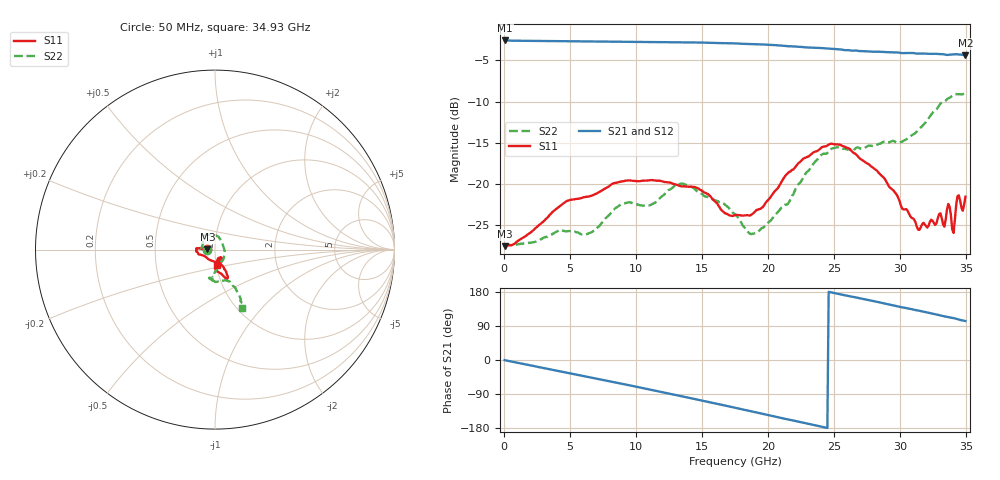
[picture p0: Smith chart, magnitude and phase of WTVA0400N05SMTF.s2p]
! 50 ohm 2-Port S-parameters measured by Modelithics Inc support@modelithics.com  Tampa, FL USA 813-866-6335 (February 2024)
! Smiths Interconnect,  4dB P/N: WTVA0400N05SMTF, Temperature: 125 C
! Board: 10 mil Rogers 4350B, Mounting Pad Dimensions: Length: 15 mils, Width: 25 mils, Gap: 40 mils.
# Hz S RI R 50
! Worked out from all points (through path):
!   352 points, 50 MHz to 34.93 GHz, reference 50 ohm
!   highest |S21| = -2.60 dB at 100 MHz (marker M1); lowest = -4.4 dB at 34.93 GHz (marker M2)
!   group delay of S21, straight-line fit = 20.5 ps
!   lowest |S11| = -27.5 dB at 50 MHz (marker M3), VSWR 1.09, Z = 46 + j0.113 ohm
!   |S11| at or under -10 dB: start of sweep to end of sweep
!   |S22| runs from -27.5 to -9.0 dB; largest |S21 - S12| = 0.0087
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5e7  -0.0421 0.00122  0.7413 -0.00433  0.7406 -0.00446  -0.042 -0.000425
1e8  -0.0427 0.000688  0.7414 -0.00973  0.7406 -0.00984  -0.0431 -0.000107
5.8715e9  -0.082 0.00756  0.5515 -0.4817  0.5505 -0.4812  -0.0461 -0.0181
8.956e9  -0.1036 0.00735  0.3322 -0.6484  0.3307 -0.6478  -0.0757 -0.00622
1.1742e10  -0.1044 -0.00969  0.0893 -0.7193  0.0874 -0.7184  -0.0674 0.0453
1.36325e10  -0.095 -0.0195  -0.0872 -0.7181  -0.0886 -0.7169  -0.0594 0.0806
1.7513e10  -0.0376 -0.0529  -0.4201 -0.5744  -0.4202 -0.5728  0.0284 0.0588
1.8508e10  -0.0141 -0.063  -0.4885 -0.5094  -0.4889 -0.5077  0.0425 0.0277
1.92045e10  0.00207 -0.0699  -0.5313 -0.4597  -0.5306 -0.4591  0.0509 0.0031
2.1493e10  0.0499 -0.1051  -0.6274 -0.2705  -0.6271 -0.2683  0.0337 -0.068
2.33835e10  0.0668 -0.1395  -0.6626 -0.1059  -0.6617 -0.1054  -0.00282 -0.1316
2.47765e10  0.07 -0.1612  -0.6599 0.0183  -0.6589 0.02  -0.0143 -0.1629
2.607e10  0.056 -0.1549  -0.636 0.125  -0.6345 0.1263  -0.0292 -0.1601
2.91545e10  0.00221 -0.0962  -0.5253 0.3472  -0.5205 0.3519  0.0188 -0.178
3.1443e10  0.0196 -0.049  -0.396 0.474  -0.3922 0.4755  0.0966 -0.1937
3.3035e10  0.0371 -0.0552  -0.2835 0.5431  -0.2776 0.5448  0.1426 -0.2719
3.33335e10  0.0253 -0.049  -0.2598 0.5524  -0.2556 0.5531  0.1412 -0.284
3.3632e10  0.0367 -0.0663  -0.2396 0.5571  -0.2338 0.5586  0.149 -0.2955
3.403e10  0.0196 -0.0466  -0.2144 0.5717  -0.2082 0.5728  0.1536 -0.3123
3.43285e10  0.022 -0.0815  -0.1845 0.5822  -0.1802 0.5825  0.1499 -0.3171
3.47265e10  0.0177 -0.0665  -0.1498 0.5877  -0.1485 0.5869  0.1452 -0.319
3.49255e10  0.00964 -0.0832  -0.1346 0.5878  -0.133 0.5866  0.1487 -0.3235
